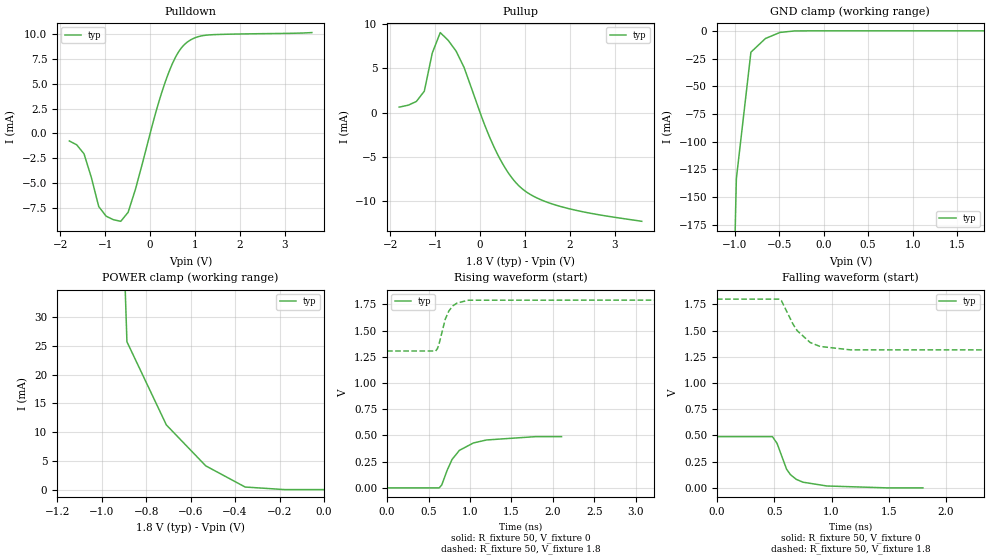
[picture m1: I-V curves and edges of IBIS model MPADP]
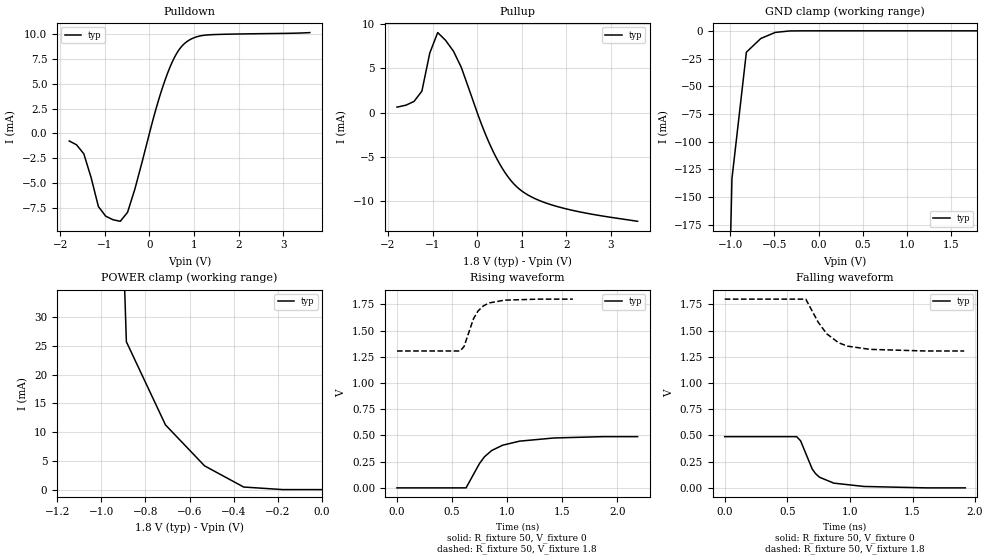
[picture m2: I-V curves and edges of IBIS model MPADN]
| Created by SiliconSmart 2008.10 (Production)
| There are several IBIS sections which it is inappropriate for this tool to
| automatically fill in - copyrights and packaging details are two examples.
| We are making it easy for you to add these things by providing commented-out
| section headers and brief descriptions of each such section.  Of course, the
| IBIS standard is the ultimate section description; these are merely summaries.
[IBIS Ver]   4.1
[File Name]   tt_1p10_1p80_25c.ibs
[File Rev]   1.0
[Date]   December 18 11:21:56
[Source]   From SiliconSmart 2008.10 (Production)
|[Notes]   Use this section for any special notes related to the file.
|   (fill in and uncomment to use this section)
|[Disclaimer]   Legal disclaimer section.
|   (fill in and uncomment to use this section)
|[Copyright]   Copyright 1995, XYZ Corp., All Rights Reserved
|   (fill in and uncomment to use this section)
[Component]   pdqs_ddr2_cl_driver_6p9ma
[Manufacturer]   Unknown
[Package]
| Variable   typ   min   max
R_pkg   18   NA   NA
L_pkg   1n   NA   NA
C_pkg   15f   NA   NA
[Pin]   signal_name   model_name   R_pin   L_pin   C_pin
1   PADP   MPADP   NA   NA   NA
2   PADN   MPADN   NA   NA   NA
3   DVSS   GND   NA   NA   NA
4   DVDD   POWER   NA   NA   NA
|[Package Model]   Package model name.  40-char limit.
|   (fill in and uncomment to use this section)
[Pin Mapping]  pulldown_ref   pullup_ref   gnd_clamp_ref  power_clamp_ref
1   DVSS   DVDD   DVSS   DVDD
2   DVSS   DVDD   DVSS   DVDD
3   DVSS   NC   NC   NC
4   NC   DVDD   NC   NC
[Diff Pin]  inv_pin  vdiff  tdelay_typ tdelay_min tdelay_max
1   2   NA   -59.67p   NA   NA
| Models and submodels in the file (2): MPADP (I/O), MPADN (I/O)
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|PADP pin
[Model]   MPADP
Model_type I/O
Polarity Non-Inverting
Vinl = 0.8
Vinh = 2.0
Vmeas = 0.9
| Capacitance   typ   min   max
C_comp   6.42p   NA   NA
| Variables   typ   min   max
[Temperature Range]   25   NA   NA
[Voltage Range]   1.8   NA   NA
[Pullup Reference]   1.8   NA   NA
[Pulldown Reference]   0.0   NA   NA
[POWER Clamp Reference]   1.8   NA   NA
[GND Clamp Reference]   0.0   NA   NA
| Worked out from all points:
|   slope of the pulldown table from 0 to 0.27 V, typ, clamps not added: 63.1 ohm
|   slope of the pullup table from 0 to 0.27 V, typ, clamps not added: 78.4 ohm
|   GND clamp passes 1 mA (typ) near -0.44 V on its own axis
|   POWER clamp passes 1 mA (typ) near -0.38 V on its own axis
|   falling waveform, R_fixture 50, V_fixture 0: 20-80 % time 138ps typ, NA min, NA max; typ from 0.489 V to 0 V
|   falling waveform, R_fixture 50, V_fixture 1.8: 20-80 % time 195ps typ, NA min, NA max; typ from 1.8 V to 1.3 V
|   rising waveform, R_fixture 50, V_fixture 0: 20-80 % time 260ps typ, NA min, NA max; typ from 0 V to 0.489 V
|   rising waveform, R_fixture 50, V_fixture 1.8: 20-80 % time 122ps typ, NA min, NA max; typ from 1.3 V to 1.8 V
[Pulldown]
| Voltage   I(typ)   I(min)   I(max)
-1.8V     -761.5uA   NA         NA
-1.473V   -2.052mA   NA         NA
-1.145V   -7.351mA   NA         NA
-981.8mV  -8.317mA   NA         NA
-654.5mV  -8.833mA   NA         NA
-490.9mV  -7.931mA   NA         NA
140.6mV   2.355mA    NA         NA
365.6mV   5.542mA    NA         NA
562.5mV   7.638mA    NA         NA
759.4mV   8.911mA    NA         NA
1.266V    9.877mA    NA         NA
3.6V      10.13mA    NA         NA
[GND Clamp]
| Voltage   I(typ)   I(min)   I(max)
-1.8V     -4.426A    NA         NA
-1.145V   -702.1mA   NA         NA
-981.8mV  -133.3mA   NA         NA
-818.2mV  -19.27mA   NA         NA
-654.5mV  -6.911mA   NA         NA
-490.9mV  -1.444mA   NA         NA
-327.3mV  -103.9uA   NA         NA
1.8V      26.57nA    NA         NA
[Pullup]
| Voltage   I(typ)   I(min)   I(max)
-1.8V     617.4uA    NA         NA
-1.418V   1.248mA    NA         NA
-1.241V   2.414mA    NA         NA
-1.064V   6.729mA    NA         NA
-886.4mV  9.041mA    NA         NA
-531.8mV  6.93mA     NA         NA
-354.5mV  5.083mA    NA         NA
309.4mV   -3.883mA   NA         NA
590.6mV   -6.529mA   NA         NA
871.9mV   -8.323mA   NA         NA
1.772V    -10.6mA    NA         NA
3.6V      -12.3mA    NA         NA
[POWER Clamp]
| Voltage   I(typ)   I(min)   I(max)
-1.8V     4.331A     NA         NA
-1.773V   4.155A     NA         NA
-1.595V   3.037A     NA         NA
-1.418V   1.962A     NA         NA
-1.241V   976.7mA    NA         NA
-1.064V   234.9mA    NA         NA
-886.4mV  25.71mA    NA         NA
-709.1mV  11.25mA    NA         NA
-531.8mV  4.13mA     NA         NA
-354.5mV  447.2uA    NA         NA
-177.3mV  4.06uA     NA         NA
0V        0A         NA         NA
[Ramp]
dV/dt_r   0.29492/0.190678n NA   NA
dV/dt_f   0.29493/0.166386n NA   NA
R_load = 50
[Falling Waveform]
R_fixture = 50
V_fixture = 0
| Time   V(typ)   V(min)   V(max)
0s        488.5mV    NA         NA
484.3ps   488.5mV    NA         NA
524.6ps   424.3mV    NA         NA
607.6ps   178.5mV    NA         NA
640.9ps   126.6mV    NA         NA
691.9ps   81.69mV    NA         NA
749.8ps   54.3mV     NA         NA
959.6ps   17.94mV    NA         NA
1.485ns   24.89uV    NA         NA
1.798ns   24.89uV    NA         NA
[Falling Waveform]
R_fixture = 50
V_fixture = 1.8
| Time   V(typ)   V(min)   V(max)
0s        1.8V       NA         NA
547.6ps   1.8V       NA         NA
561.7ps   1.788V     NA         NA
663.7ps   1.562V     NA         NA
701.6ps   1.498V     NA         NA
814.1ps   1.386V     NA         NA
899.4ps   1.349V     NA         NA
1.165ns   1.316V     NA         NA
31.56ns   1.305V     NA         NA
[Rising Waveform]
R_fixture = 50
V_fixture = 0
| Time   V(typ)   V(min)   V(max)
0s        24.6uV     NA         NA
629.1ps   24.6uV     NA         NA
659.3ps   27.87mV    NA         NA
724.8ps   168.4mV    NA         NA
783.7ps   270.9mV    NA         NA
871.5ps   357.3mV    NA         NA
1.041ns   428.4mV    NA         NA
1.199ns   456.7mV    NA         NA
1.791ns   488.5mV    NA         NA
2.103ns   488.5mV    NA         NA
[Rising Waveform]
R_fixture = 50
V_fixture = 1.8
| Time   V(typ)   V(min)   V(max)
0s        1.305V     NA         NA
585.8ps   1.305V     NA         NA
606ps     1.327V     NA         NA
624.6ps   1.365V     NA         NA
702.4ps   1.611V     NA         NA
746.2ps   1.689V     NA         NA
796.1ps   1.737V     NA         NA
844.5ps   1.763V     NA         NA
981.2ps   1.79V      NA         NA
31.56ns   1.8V       NA         NA
|PADN pin
[Model]   MPADN
Model_type I/O
Polarity Inverting
Vinl = 0.8
Vinh = 2.0
Vmeas = 0.9
| Capacitance   typ   min   max
C_comp   6.42p   NA   NA
| Variables   typ   min   max
[Temperature Range]   25   NA   NA
[Voltage Range]   1.8   NA   NA
[Pullup Reference]   1.8   NA   NA
[Pulldown Reference]   0.0   NA   NA
[POWER Clamp Reference]   1.8   NA   NA
[GND Clamp Reference]   0.0   NA   NA
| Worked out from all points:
|   slope of the pulldown table from 0 to 0.27 V, typ, clamps not added: 63.1 ohm
|   slope of the pullup table from 0 to 0.27 V, typ, clamps not added: 78.4 ohm
|   GND clamp passes 1 mA (typ) near -0.44 V on its own axis
|   POWER clamp passes 1 mA (typ) near -0.38 V on its own axis
|   falling waveform, R_fixture 50, V_fixture 0: 20-80 % time 138ps typ, NA min, NA max; typ from 0.489 V to 0 V
|   falling waveform, R_fixture 50, V_fixture 1.8: 20-80 % time 195ps typ, NA min, NA max; typ from 1.8 V to 1.3 V
|   rising waveform, R_fixture 50, V_fixture 0: 20-80 % time 249ps typ, NA min, NA max; typ from 0 V to 0.489 V
|   rising waveform, R_fixture 50, V_fixture 1.8: 20-80 % time 123ps typ, NA min, NA max; typ from 1.3 V to 1.8 V
[Pulldown]
| Voltage   I(typ)   I(min)   I(max)
-1.8V     -761.5uA   NA         NA
-1.473V   -2.052mA   NA         NA
-1.145V   -7.351mA   NA         NA
-981.8mV  -8.317mA   NA         NA
-654.5mV  -8.833mA   NA         NA
-490.9mV  -7.931mA   NA         NA
140.6mV   2.355mA    NA         NA
365.6mV   5.542mA    NA         NA
562.5mV   7.638mA    NA         NA
759.4mV   8.911mA    NA         NA
1.266V    9.877mA    NA         NA
3.6V      10.13mA    NA         NA
[GND Clamp]
| Voltage   I(typ)   I(min)   I(max)
-1.8V     -4.426A    NA         NA
-1.145V   -702.1mA   NA         NA
-981.8mV  -133.3mA   NA         NA
-818.2mV  -19.27mA   NA         NA
-654.5mV  -6.911mA   NA         NA
-490.9mV  -1.444mA   NA         NA
-327.3mV  -103.9uA   NA         NA
1.8V      26.57nA    NA         NA
[Pullup]
| Voltage   I(typ)   I(min)   I(max)
-1.8V     617.4uA    NA         NA
-1.418V   1.248mA    NA         NA
-1.241V   2.414mA    NA         NA
-1.064V   6.729mA    NA         NA
-886.4mV  9.041mA    NA         NA
-531.8mV  6.93mA     NA         NA
-354.5mV  5.083mA    NA         NA
309.4mV   -3.883mA   NA         NA
590.6mV   -6.529mA   NA         NA
871.9mV   -8.323mA   NA         NA
1.772V    -10.6mA    NA         NA
3.6V      -12.3mA    NA         NA
[POWER Clamp]
| Voltage   I(typ)   I(min)   I(max)
-1.8V     4.331A     NA         NA
-1.773V   4.155A     NA         NA
-1.595V   3.037A     NA         NA
-1.418V   1.962A     NA         NA
-1.241V   976.7mA    NA         NA
-1.064V   234.9mA    NA         NA
-886.4mV  25.71mA    NA         NA
-709.1mV  11.25mA    NA         NA
-531.8mV  4.13mA     NA         NA
-354.5mV  447.2uA    NA         NA
-177.3mV  4.06uA     NA         NA
0V        0A         NA         NA
[Ramp]
dV/dt_r   0.294921/0.186317n NA   NA
dV/dt_f   0.29493/0.166573n NA   NA
R_load = 50
[Falling Waveform]
R_fixture = 50
V_fixture = 0
| Time   V(typ)   V(min)   V(max)
0s        488.5mV    NA         NA
574.4ps   488.5mV    NA         NA
605.9ps   449.1mV    NA         NA
698.5ps   180.1mV    NA         NA
724.8ps   136.5mV    NA         NA
757.2ps   101.1mV    NA         NA
871.5ps   44.96mV    NA         NA
1.112ns   13.35mV    NA         NA
1.609ns   25.08uV    NA         NA
1.922ns   25.08uV    NA         NA
[Falling Waveform]
R_fixture = 50
V_fixture = 1.8
| Time   V(typ)   V(min)   V(max)
0s        1.8V       NA         NA
647.3ps   1.8V       NA         NA
746.2ps   1.581V     NA         NA
814.1ps   1.47V      NA         NA
910ps     1.384V     NA         NA
981.2ps   1.351V     NA         NA
1.159ns   1.321V     NA         NA
1.601ns   1.305V     NA         NA
1.913ns   1.305V     NA         NA
[Rising Waveform]
R_fixture = 50
V_fixture = 0
| Time   V(typ)   V(min)   V(max)
0s        24.59uV    NA         NA
627.1ps   24.59uV    NA         NA
749.8ps   233.3mV    NA         NA
794.7ps   296.8mV    NA         NA
860.4ps   356.5mV    NA         NA
959.6ps   406.9mV    NA         NA
1.113ns   445.4mV    NA         NA
1.426ns   475.9mV    NA         NA
1.872ns   488.5mV    NA         NA
2.185ns   488.5mV    NA         NA
[Rising Waveform]
R_fixture = 50
V_fixture = 1.8
| Time   V(typ)   V(min)   V(max)
0s        1.305V     NA         NA
573.1ps   1.305V     NA         NA
609ps     1.348V     NA         NA
694.2ps   1.612V     NA         NA
735.5ps   1.686V     NA         NA
785.6ps   1.736V     NA         NA
838.5ps   1.764V     NA         NA
974.6ps   1.79V      NA         NA
1.284ns   1.8V       NA         NA
1.597ns   1.8V       NA         NA
